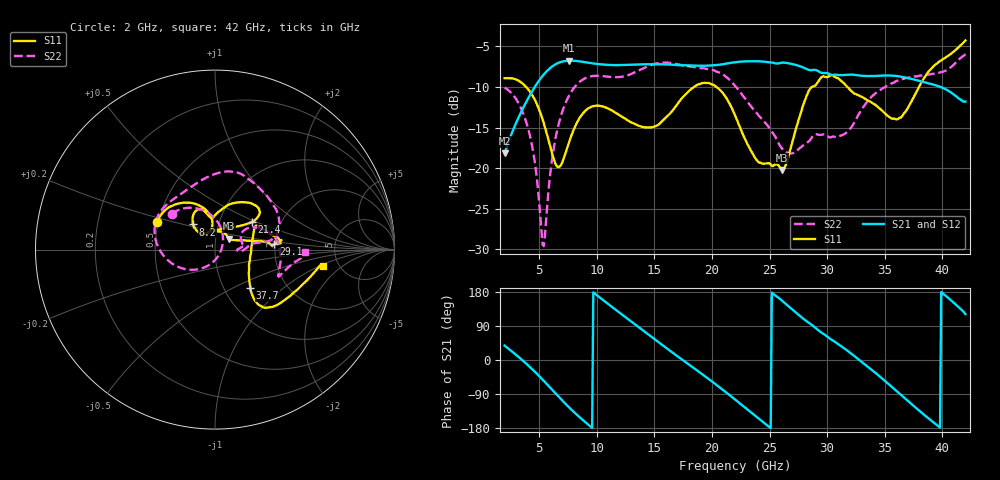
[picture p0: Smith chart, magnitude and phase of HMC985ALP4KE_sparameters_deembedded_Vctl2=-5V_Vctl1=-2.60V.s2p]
!s2p File: Measurements: S11, S21, S12, S22
# GHz S dB R 50.0
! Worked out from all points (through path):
!   401 points, 2 GHz to 42 GHz, reference 50 ohm
!   highest |S21| = -6.76 dB at 7.6 GHz (marker M1); lowest = -18.2 dB at 2 GHz (marker M2)
!   lowest |S11| = -20.2 dB at 26.1 GHz (marker M3), VSWR 1.22, Z = 57.7 + j7.11 ohm
!   |S11| at or under -10 dB: 3.864 GHz to 18.46 GHz (14.59 GHz wide, 131 % of centre); 20.37 GHz to 28.68 GHz (8.31 GHz wide, 33.9 % of centre); 31.76 GHz to 37.97 GHz (6.214 GHz wide, 17.8 % of centre)
!   |S22| runs from -29.6 to -6.0 dB; largest |S21 - S12| = 0.00052
!   S11 on the Smith chart (normalised r, x): 2 GHz: 0.49, +0.17; 8.2 GHz: 0.76, +0.22; 21.4 GHz: 1.43, +0.48; 29.1 GHz: 1.97, +0.14; 37.7 GHz: 1.33, -0.62; 42 GHz: 3.79, -1.12
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2  -8.93 154.6  -18.18 37.9  -18.19 37.9  -10.06 140.3
4.1  -10.39 120.0  -11.26 -15.8  -11.26 -15.8  -15.44 89.0
5.4  -14.47 97.7  -8.46 -55.1  -8.47 -55.1  -29.62 -34.5
6.6  -19.85 112.4  -7.08 -94.1  -7.08 -94.1  -15.12 -140.1
7.6  -16.80 133.9  -6.76 -125.2  -6.77 -125.2  -11.05 -170.6
8.2  -14.63 131.0  -6.80 -142.5  -6.81 -142.5  -9.81 175.1
8.7  -13.44 126.1  -6.89 -156.1  -6.89 -156.1  -9.17 165.1
10.4  -12.37 110.7  -7.23 161.6  -7.23 161.6  -8.65 140.1
12.4  -13.85 102.5  -7.30 115.1  -7.30 115.1  -8.68 115.2
15.4  -14.60 91.2  -7.22 46.1  -7.23 46.1  -7.06 78.6
18.2  -10.27 59.5  -7.36 -16.2  -7.36 -16.2  -7.50 53.5
21.4  -11.74 36.9  -7.09 -89.5  -7.09 -89.5  -8.96 13.8
22  -13.46 40.6  -6.96 -104.2  -6.96 -104.2  -9.85 10.1
24.2  -19.34 86.9  -6.85 -157.9  -6.85 -157.9  -13.75 8.3
26.1  -20.24 38.8  -7.01 156.2  -7.01 156.2  -17.62 -3.0
28.7  -9.98 4.1  -7.92 91.9  -7.93 91.9  -16.15 6.1
29.1  -9.61 5.5  -7.96 81.6  -7.97 81.6  -15.83 5.2
32.4  -10.85 24.3  -8.52 9.5  -8.52 9.5  -14.27 33.6
35.4  -13.70 6.9  -8.59 -65.3  -8.60 -65.3  -9.73 14.6
37.7  -10.77 -47.3  -9.14 -126.2  -9.14 -126.1  -8.69 -6.0
39.7  -6.91 -45.0  -9.93 -176.0  -9.93 -175.9  -8.27 -22.7
42  -4.28 -8.7  -11.80 121.1  -11.81 121.2  -5.96 -1.7
